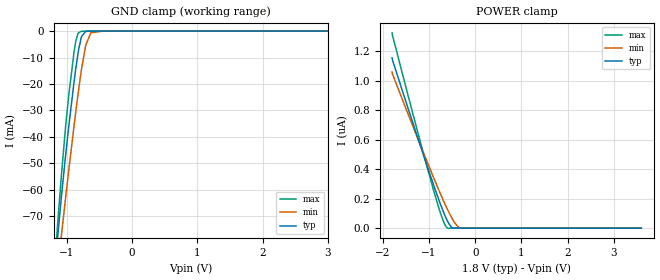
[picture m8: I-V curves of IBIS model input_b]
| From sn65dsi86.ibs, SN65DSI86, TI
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|   Model
[Model]   input_b
Model_type   Input
Vinl = 0.54
Vinh = 1.26
|   typ   min   max
C_comp   1.133pF   1.092pF   1.183pF
[Voltage Range]   1.8   1.65   1.98
[Temperature Range]   27   125   -40
[Power Clamp Reference]   1.8   1.65   1.98
[GND Clamp Reference]   -0   -0   -0
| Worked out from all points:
|   GND clamp passes 1 mA (typ) near -0.74 V on its own axis
[GND Clamp]
|   Voltage   I(typ)   I(min)   I(max)
-1.8V     -308mA     -294.7mA   -317.4mA
-1.217V   -100.4mA   -108.4mA   -98.82mA
-1.141V   -77.87mA   -90.3mA    -72.89mA
-1.087V   -63.42mA   -77.98mA   -55.59mA
-1.028V   -48.94mA   -64.84mA   -38.42mA
-968.4mV  -35.52mA   -52.05mA   -23.65mA
-887.4mV  -18.7mA    -35.25mA   -7.366mA
-817.2mV  -6.639mA   -21.68mA   -578.5uA
-774mV    -2.027mA   -14.15mA   -80.69uA
-714.6mV  -173.1uA   -5.777mA   -5.695uA
-633.6mV  -4.369uA   -642.7uA   -123nA
3.595V    0A         0A         0A
[POWER Clamp]
|   Voltage   I(typ)   I(min)   I(max)
-1.8V     1.155uA    1.059uA    1.324uA
-1.795V   1.142uA    1.047uA    1.311uA
-1.465V   822.6nA    782.6nA    912.6nA
-930.6mV  318.3nA    364.4nA    288nA
-757.8mV  166.2nA    235.9nA    105.5nA
-682.2mV  105nA      182nA      40.12nA
-617.4mV  58.08nA    137.7nA    4.968nA
-531mV    12.14nA    83.04nA    0A
-487.8mV  355.5pA    58.57nA    0A
-396mV    0A         17.53nA    0A
-315mV    0A         0A         0A
3.595V    0A         0A         0A
